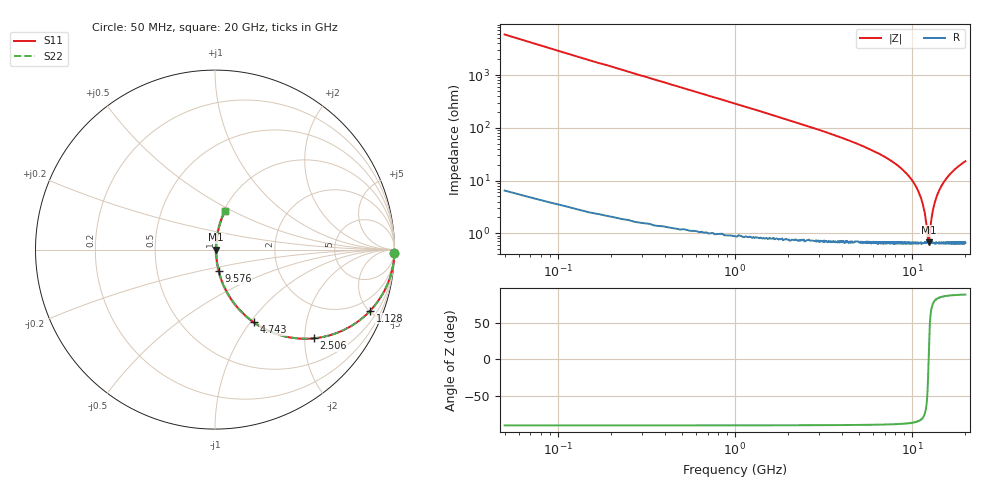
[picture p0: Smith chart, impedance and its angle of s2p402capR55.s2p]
! AVX Thin Film Operation		Date: September 2011
! Description: Accu-P® Series, Thin Film, SMD, RF Capacitor
! Part Number: 04021JR55ZBW/STR
! 50 MHz  -  20 GHz
! Serial Measurements
# MHZ S MA R 50
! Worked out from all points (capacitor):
!   1000 points, 50 MHz to 20 GHz, reference 50 ohm
!   read as one part in series: C = 550 fF near 149.8 MHz
!   lowest |Z| = 680 mohm at 12.39 GHz (marker M1)
!   series resonance near 12.39 GHz, so ESL is about 300 pH
!   S11 on the Smith chart (normalised r, x): 50 MHz: open; 1.128 GHz: 1.01, -5.09; 2.506 GHz: 1.01, -2.22; 4.743 GHz: 1.01, -1.04; 9.576 GHz: 1.01, -0.24; 20 GHz: 1.01, +0.46
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50  1 -1.0  0.017 88.9  0.017 88.9  1 -1.0
229.73  0.997 -4.5  0.079 85.4  0.079 85.4  0.997 -4.5
409.459  0.99 -8.1  0.14 81.8  0.14 81.8  0.99 -8.1
709.009  0.971 -13.8  0.239 76.1  0.239 76.1  0.971 -13.8
1128.378  0.93 -21.4  0.366 68.4  0.366 68.4  0.93 -21.4
2506.306  0.74 -41.9  0.668 47.7  0.668 47.7  0.74 -41.9
3384.985  0.618 -51.3  0.781 38.2  0.781 38.2  0.618 -51.3
4742.943  0.459 -61.9  0.882 27.4  0.882 27.4  0.459 -61.9
6700  0.291 -71.9  0.951 16.9  0.951 16.9  0.291 -71.9
9575.676  0.12 -80.0  0.986 6.9  0.986 6.9  0.12 -80.0
10034.99  0.098 -80.6  0.989 5.6  0.989 5.6  0.098 -80.6
10913.66  0.059 -80.3  0.992 3.4  0.992 3.4  0.059 -80.3
11492.79  0.036 -77.5  0.993 2.0  0.993 2.0  0.036 -77.5
11892.19  0.02 -70.1  0.993 1.1  0.993 1.1  0.02 -70.1
12291.59  0.007529 -30.1  0.993 0.2  0.993 0.2  0.007529 -30.1
12391.44  0.006501 -0.4  0.993 0.0  0.993 0.0  0.006501 -0.4
12511.26  0.007861 34.0  0.993 -0.3  0.993 -0.3  0.007861 34.0
12890.69  0.019 69.4  0.993 -1.0  0.993 -1.0  0.019 69.4
13350  0.035 77.4  0.993 -2.0  0.993 -2.0  0.035 77.4
14608.11  0.077 80.8  0.991 -4.4  0.991 -4.4  0.077 80.8
16684.99  0.139 79.4  0.984 -8.0  0.984 -8.0  0.139 79.4
20000  0.225 75.4  0.968 -13.0  0.968 -13.0  0.225 75.4
